FUNCTION_BLOCK FB_DO_IED_LD1_MMXU1_NamPlt EXTENDS FB_AcsiCommonDataClass
VAR_INPUT
	vendor: FB_AcsiDATypeVisString255 := (fc:=ACSI_FC_DC, sValue:='Beckhoff Automation', bLinkResult:=THIS^.AddDataToContainer(ipData:=vendor));
	swRev: FB_AcsiDATypeVisString255 := (fc:=ACSI_FC_DC, sValue:='1.0', bLinkResult:=THIS^.AddDataToContainer(ipData:=swRev));
	d: FB_AcsiDATypeVisString255 := (fc:=ACSI_FC_DC, sValue:='Demo measured value', bLinkResult:=THIS^.AddDataToContainer(ipData:=d));
	configRev: FB_AcsiDATypeVisString255 := (fc:=ACSI_FC_DC, sValue:='1', bLinkResult:=THIS^.AddDataToContainer(ipData:=configRev));
	ldNs: FB_AcsiDATypeVisString255 := (fc:=ACSI_FC_EX, sValue:='IEC 61850-7-4:2007', bLinkResult:=THIS^.AddDataToContainer(ipData:=ldNs));
END_VAR
VAR
END_VAR

END_FUNCTION_BLOCK
